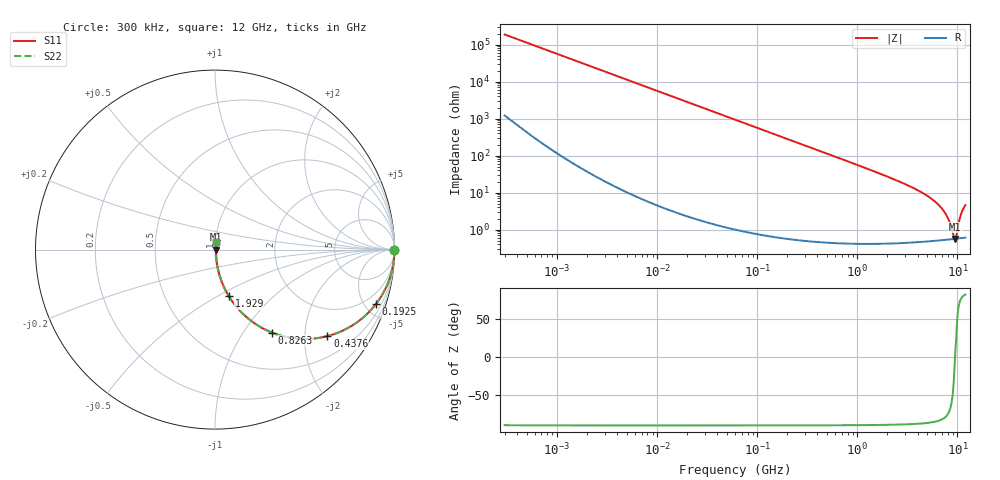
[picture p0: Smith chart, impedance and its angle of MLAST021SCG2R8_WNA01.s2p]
! MLAST021SCG2R8_WNA01  S-PARAMETER MODEL  ( General Type )
! Model Generated by TAIYO YUDEN Corporation (http://www.ty-top.com)
! Version 1.0
! TAIYO YUDEN Control No. 220901
! Copyright(c) 2022 TAIYO YUDEN CO.,LTD. All Rights Reserved.
! Product Description (link to TY-COMPAS)
! https://ds.yuden.co.jp/TYCOMPAS/or/detail?pn=MLAST021SCG2R8BWNA01&u=M
! Products Name : Multilayer Ceramic Capacitors
! Characteristics :
!  Capacitance : 2.8 pF , Rated Voltage : 25V , TCC : CG / C0G
!  Case Size : 0.25 x 0.125 / 0.0098 x 0.0049 [mm/inch] , Thickness : 0.125 / 0.0049 [mm/inch]
!  (Conditions: Temperature = 25 degC , DC Bias Current/Voltage = 0A / 0V)
! External Node Assignments :
!  1  o---| |---o  2
! GND o---------o GND
! Frequency Range : 0.3MHz  -  12000MHz  [ 401 STEP ]
# MHz S RI R 50
! Freq[MHz].  S11 Real  S11 Imag  S21 Real  S21 Imag  S12 Real  S12 Imag  S22 Real  S22 Imag
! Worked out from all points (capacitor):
!   401 points, 300 kHz to 12 GHz, reference 50 ohm
!   read as one part in series: C = 2.8 pF near 316.3 kHz
!   lowest |Z| = 565 mohm at 9.454 GHz (marker M1)
!   series resonance near 9.454 GHz, so ESL is about 100 pH
!   S11 on the Smith chart (normalised r, x): 300 kHz: open; 192.5 MHz: 1.01, -5.90; 437.6 MHz: 1.01, -2.59; 826.3 MHz: 1.01, -1.37; 1.929 GHz: 1.01, -0.56; 12 GHz: 1.01, +0.09
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0.3  1 -0.000528  3.67e-06 0.000528  3.67e-06 0.000528  1 -0.000528
1.769972  1 -0.00311  1.4e-05 0.00311  1.4e-05 0.00311  1 -0.00311
10.44266  0.9996 -0.0184  0.000352 0.0184  0.000352 0.0184  0.9996 -0.0184
60  0.9889 -0.1044  0.0111 0.1044  0.0111 0.1044  0.9889 -0.1044
192.4766  0.8966 -0.3035  0.1034 0.3035  0.1034 0.3035  0.8966 -0.3035
353.9943  0.7194 -0.4478  0.2806 0.4478  0.2806 0.4478  0.7194 -0.4478
437.5599  0.6265 -0.482  0.3735 0.482  0.3735 0.482  0.6265 -0.482
826.3444  0.3189 -0.463  0.6811 0.463  0.6811 0.463  0.3189 -0.463
1262.535  0.1659 -0.3673  0.8341 0.3673  0.8341 0.3673  0.1659 -0.3673
1928.972  0.0772 -0.2595  0.9228 0.2595  0.9228 0.2595  0.0772 -0.2595
2088.533  0.0662 -0.2407  0.9338 0.2407  0.9338 0.2407  0.0662 -0.2407
3944.255  0.0183 -0.1164  0.9817 0.1164  0.9817 0.1164  0.0183 -0.1164
6026.253  0.00806 -0.0553  0.9919 0.0553  0.9919 0.0553  0.00806 -0.0553
6879.757  0.00663 -0.0385  0.9934 0.0385  0.9934 0.0385  0.00663 -0.0385
7648.807  0.00594 -0.0255  0.9941 0.0255  0.9941 0.0255  0.00594 -0.0255
8281.503  0.00566 -0.0159  0.9943 0.0159  0.9943 0.0159  0.00566 -0.0159
8966.534  0.00557 -0.0064  0.9944 0.0064  0.9944 0.0064  0.00557 -0.0064
9454.42  0.00562 -2.72e-07  0.9944 2.72e-07  0.9944 2.72e-07  0.00562 -2.72e-07
9968.853  0.00576 0.00745  0.9942 -0.00745  0.9942 -0.00745  0.00576 0.00745
10511.28  0.00614 0.0184  0.9939 -0.0184  0.9939 -0.0184  0.00614 0.0184
11083.22  0.00678 0.0297  0.9932 -0.0297  0.9932 -0.0297  0.00678 0.0297
12000  0.00809 0.0451  0.9919 -0.0451  0.9919 -0.0451  0.00809 0.0451
